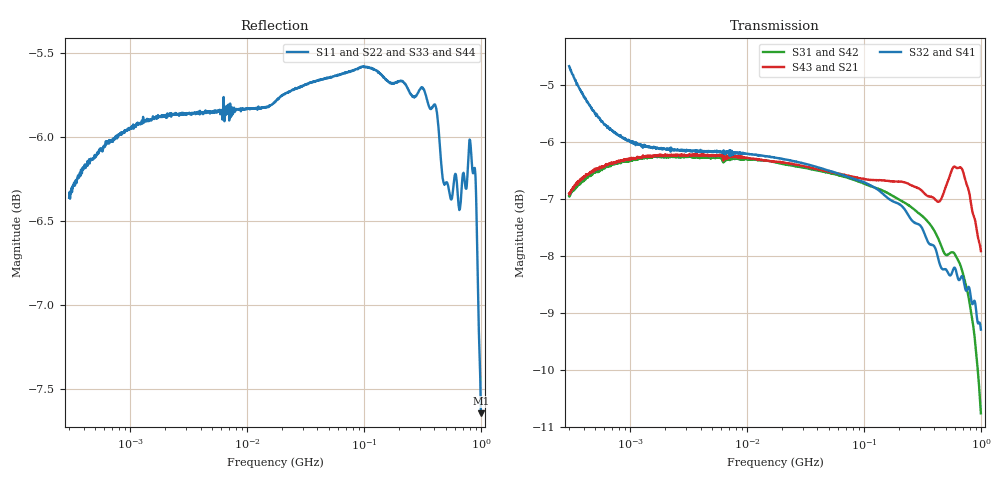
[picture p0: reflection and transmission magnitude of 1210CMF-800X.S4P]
!s-Parameter Generated by FASTRON Sdn. Bhd.
!FASTRON P/N : 1210CMF-800X
!Keysight Technologies: E5071C_MY46733604_B.14.02
!Date: Mon Mar 09 14:45:32 2026
!Version  :Rev00  Mon Mar 09 14:45:32 2026
!Data & Calibration Information:
!Freq	S11:SOLT4(ON)	S12:SOLT4(ON)	S13:SOLT4(ON)	S14:SOLT4(ON)
!	S21:SOLT4(ON)	S22:SOLT4(ON)	S23:SOLT4(ON)	S24:SOLT4(ON)
!	S31:SOLT4(ON)	S32:SOLT4(ON)	S33:SOLT4(ON)	S34:SOLT4(ON)
!	S41:SOLT4(ON)	S42:SOLT4(ON)	S43:SOLT4(ON)	S44:SOLT4(ON)
!PortZ  Port1:50+j0  Port2:50+j0  Port3:50+j0  Port4:50+j0
!When reading reference impedance value at option line is always used.
! Remarks : This data is being provided solely for informational purposes.
# Hz S dB R 50
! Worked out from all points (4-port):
!   1601 points, 300 kHz to 1 GHz, reference 50 ohm
!   strongest paths, dB at 300 kHz, 2.303 MHz, 17.55 MHz, 132.8 MHz, 1 GHz:
!     S32: -4.7, -6.1, -6.3, -6.8, -9.3
!     S41: -4.6, -6.2, -6.3, -6.9, -9.7
!     S43: -6.9, -6.2, -6.3, -6.7, -7.9
!     S31: -6.9, -6.2, -6.4, -6.8, -10.8
!     S42: -6.9, -6.2, -6.4, -6.9, -10.2
!     S21: -7.0, -6.3, -6.4, -6.7, -6.4
!   lowest |S11| = -7.6 dB at 1 GHz (marker M1), VSWR 2.42, Z = 120 + j8.68 ohm
!   |S11| at or under -10 dB: nowhere
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300000  -6.36 18.6  -6.98 21.2  -6.97 -158.9  -4.73 -16.8
        -6.97 21.0  -6.36 19.0  -4.67 -16.9  -7.01 -158.6
        -6.95 -158.9  -4.67 -16.9  -6.36 19.0  -7.03 21.3
        -4.65 -17.2  -6.92 -159.0  -6.90 20.8  -6.42 19.8
3445924  -5.86 1.9  -6.25 1.6  -6.23 -179.3  -6.19 -3.3
         -6.27 1.6  -5.87 1.9  -6.12 -3.3  -6.26 -179.4
         -6.25 -179.5  -6.16 -3.3  -5.86 1.9  -6.25 1.5
         -6.18 -3.2  -6.26 -179.3  -6.22 1.7  -5.86 1.9
6.293603e7  -5.62 -1.5  -6.60 -1.2  -6.57 161.3  -6.56 -18.2
            -6.61 -1.1  -5.60 -1.6  -6.55 -18.7  -6.64 161.8
            -6.59 161.2  -6.57 -18.7  -5.60 -1.8  -6.59 -1.0
            -6.55 -18.2  -6.62 161.6  -6.56 -1.1  -5.60 -1.0
1.63161e8  -5.67 -5.4  -6.73 -0.4  -6.89 134.3  -6.96 -43.7
           -6.74 -0.4  -5.58 -5.5  -6.98 -44.9  -6.98 135.7
           -6.91 134.4  -7.00 -44.9  -5.63 -6.2  -6.71 -0.2
           -6.95 -43.8  -6.97 135.7  -6.68 -0.2  -5.60 -4.2
3.335246e8  -5.74 -8.2  -6.91 0.5  -7.32 91.0  -7.58 -86.7
            -6.94 0.5  -5.66 -8.5  -7.62 -88.5  -7.43 93.0
            -7.35 91.0  -7.64 -88.6  -5.78 -9.3  -6.92 0.5
            -7.58 -86.6  -7.43 93.0  -6.91 0.3  -5.61 -5.7
6.63301e8  -6.42 -2.2  -6.83 1.5  -8.14 13.1  -8.25 -171.0
           -6.84 1.6  -5.97 -1.2  -8.41 -169.2  -8.32 13.2
           -8.14 13.1  -8.41 -169.3  -6.60 -0.1  -6.46 1.5
           -8.27 -171.0  -8.30 13.2  -6.44 1.5  -6.56 -1.9
1e9  -7.65 4.1  -6.44 6.9  -10.79 -66.5  -9.74 103.4
     -6.45 7.1  -6.51 5.8  -9.32 112.1  -10.23 -71.8
     -10.76 -66.5  -9.29 111.9  -5.49 7.7  -7.95 3.1
     -9.71 103.2  -10.17 -71.7  -7.91 3.5  -5.84 11.7
